(* Logix 5000 AddOnInstructionDefinition export YAI_Assy_72_73_120_EIP_Hz; software revision 21.03 *)

ADD_ON_INSTRUCTION YAI_Assy_72_73_120_EIP_Hz   (* revision 1.0, vendor Yaskawa America, Inc. *)
// YAI Assembly 72/73 and 120
// Help:
// This add-on instruction is for use with input assemblie 72/73 and output assemblies 120.
// Node_Input_Assy is defined as the node's input assembly integer array.
// Node_Output_Assy is defined as the node's output assembly integer array.
// Torque limit/reference, torque compensation and torque output variables are only available with A1000.
VAR_IN_OUT
   Node_Input_Assy : AB:ETHERNET_MODULE_INT_6Bytes:I:0; {required}   // Input assembly words
   Node_Output_Assy : AB:ETHERNET_MODULE_INT_24Bytes:O:0; {required}   // Output assembly words
END_VAR
VAR_INPUT
   RunFwd : BOOL; {visible}   // Forward run command
   RunRev : BOOL; {visible}   // Reverse run command
   MFI_3 : BOOL; {visible}   // Multi-function input 3
   MFI_4 : BOOL; {visible}   // Multi-function input 4
   MFI_5 : BOOL; {visible}   // Multi-function input 5
   MFI_6 : BOOL; {visible}   // Multi-function input 6
   MFI_7 : BOOL; {visible}   // Multi-function input 7
   MFI_8 : BOOL; {visible}   // Multi-function input 8
   External_Fault : BOOL;   // External fault command (EF0)
   FaultReset : BOOL; {visible}   // Fault reset command
   MFO_1 : BOOL; {visible}   // Multi-function output (M1-M2 for A/P1000, MA/MB/MC for V1000)
   MFO_2 : BOOL; {visible}   // Multi-function output (M3-M4 for A/P1000, P1 for V1000)
   MFO_3 : BOOL; {visible}   // Multi-function output (M5-M6 for A/P1000, P2 for V1000)
   Freq_Ref : REAL; {visible}   // Frequency reference command in Hz (xx.xx resolution)
   Digital_Output_Fault_Enable : BOOL;   // Bit to enable control of fault output relay over the network
   Custom_Out_1 : INT;
   Custom_Out_2 : INT;
   Custom_Out_3 : INT;
   Custom_Out_4 : INT;
   Custom_Out_5 : INT;
   Custom_Out_6 : INT;
   Custom_Out_7 : INT;
   Custom_Out_8 : INT;
   Custom_Out_9 : INT;
   Custom_Out_10 : INT;
END_VAR
VAR_OUTPUT
   Faulted : BOOL; {access Read Only, visible}   // Drive faulted status bit
   Output_Freq : REAL; {access Read Only, visible}   // Drive output frequency in Hz (xx.xx resolution)
   RunningFwd : BOOL; {access Read Only, visible}   // Drive running forward status bit
   Faulted1 : BOOL; {access Read Only, visible}   // Drive faulted status bit
   NetCtrlStatus : BOOL; {access Read Only, visible}   // Drive network run source status bit (1 = source coming from network)
   NetRefStatus : BOOL; {access Read Only, visible}   // Drive network reference status bit (1 = reference coming from network)
   Output_Freq1 : REAL; {access Read Only, visible}   // Drive output frequency in Hz (xx.xx resolution)
   Ready : BOOL; {access Read Only, visible}   // Drive ready status bit
   RunningFwd1 : BOOL; {access Read Only, visible}   // Drive running forward status bit
   RunningRev : BOOL; {access Read Only, visible}   // Drive running reverse status bit
   Torque_Actual : REAL; {access Read Only, visible}   // Drive torque output in engineering units.
   Warning : BOOL; {access Read Only, visible}   // Drive warning (alarm) status bit
   At_Speed : BOOL; {access Read Only, visible}   // Drive at commanded speed status bit
   Drive_State : INT; {access Read Only}   // Drive Status - Refer to class 0x29, Instance 0x1, Attribute 0x6 for details
END_VAR
VAR_INPUT
   Motor_Rated_Torq : REAL := 100.0; {visible}   // Motor rated torque (Engineering units)
END_VAR
VAR
   FRef_Convert : DINT;
   FOut_Convert : REAL;
   FOut_Temp : REAL;
   TRef_Convert : INT;
   TComp_Convert : INT;
   TOut_Convert : REAL;
   TOut_Temp : REAL;
   IOut_Temp : REAL;
   IOut_Convert : REAL;
   AO1_Convert : INT;
   AO2_Convert : INT;
   Motor_Speed_Temp : REAL;
   Motor_Speed_Convert : REAL;
   Freq_Cmd_Temp : REAL;
   Freq_Cmd_Convert : REAL;
   AI1_Temp : REAL;
   AI1_Convert : REAL;
   AI2_Temp : REAL; {access None}
   AI2_Convert : REAL; {access None}
   AI3_Temp : REAL; {access None}
   AI3_Convert : REAL; {access None}
   DriveStatusTempBits : INT;
   Tout_Convert_Temp : REAL;
END_VAR

ROUTINE Logic   (* ladder *)
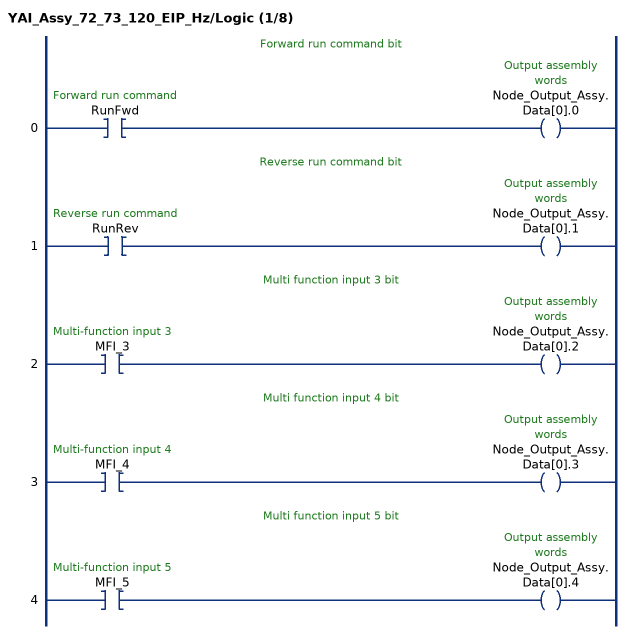
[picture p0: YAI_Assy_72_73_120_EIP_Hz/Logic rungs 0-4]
   // Forward run command bit
   0: XIC(RunFwd)OTE(Node_Output_Assy.Data[0].0);
   // Reverse run command bit
   1: XIC(RunRev)OTE(Node_Output_Assy.Data[0].1);
   // Multi function input 3 bit
   2: XIC(MFI_3)OTE(Node_Output_Assy.Data[0].2);
   // Multi function input 4 bit
   3: XIC(MFI_4)OTE(Node_Output_Assy.Data[0].3);
   // Multi function input 5 bit
   4: XIC(MFI_5)OTE(Node_Output_Assy.Data[0].4);
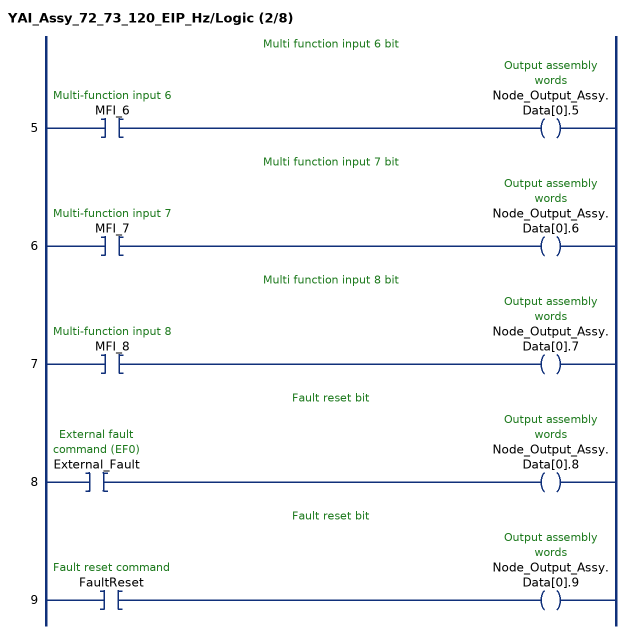
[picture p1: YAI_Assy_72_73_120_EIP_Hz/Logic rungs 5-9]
   // Multi function input 6 bit
   5: XIC(MFI_6)OTE(Node_Output_Assy.Data[0].5);
   // Multi function input 7 bit
   6: XIC(MFI_7)OTE(Node_Output_Assy.Data[0].6);
   // Multi function input 8 bit
   7: XIC(MFI_8)OTE(Node_Output_Assy.Data[0].7);
   // Fault reset bit
   8: XIC(External_Fault)OTE(Node_Output_Assy.Data[0].8);
   // Fault reset bit
   9: XIC(FaultReset)OTE(Node_Output_Assy.Data[0].9);
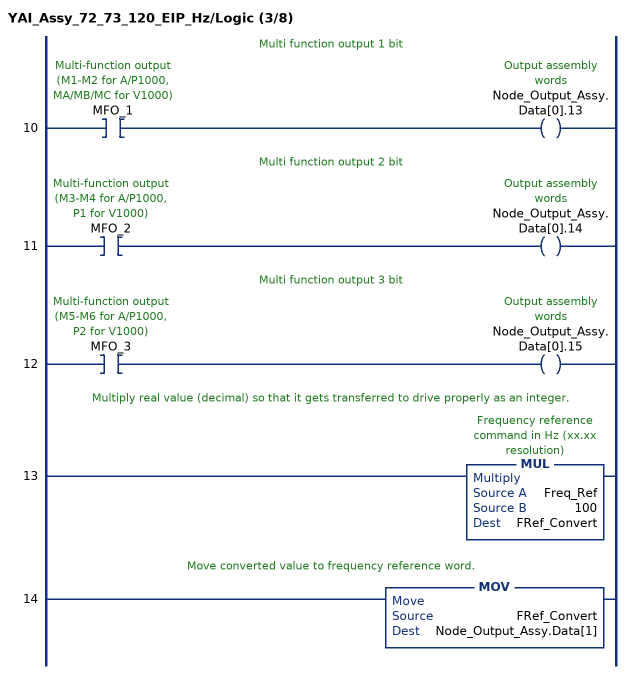
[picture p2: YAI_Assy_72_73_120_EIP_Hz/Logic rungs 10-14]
   // Multi function output 1 bit
   10: XIC(MFO_1)OTE(Node_Output_Assy.Data[0].13);
   // Multi function output 2 bit
   11: XIC(MFO_2)OTE(Node_Output_Assy.Data[0].14);
   // Multi function output 3 bit
   12: XIC(MFO_3)OTE(Node_Output_Assy.Data[0].15);
   // Multiply real value (decimal) so that it gets transferred to drive properly as an integer.
   13: MUL(Freq_Ref,100,FRef_Convert);
   // Move converted value to frequency reference word.
   14: MOV(FRef_Convert,Node_Output_Assy.Data[1]);
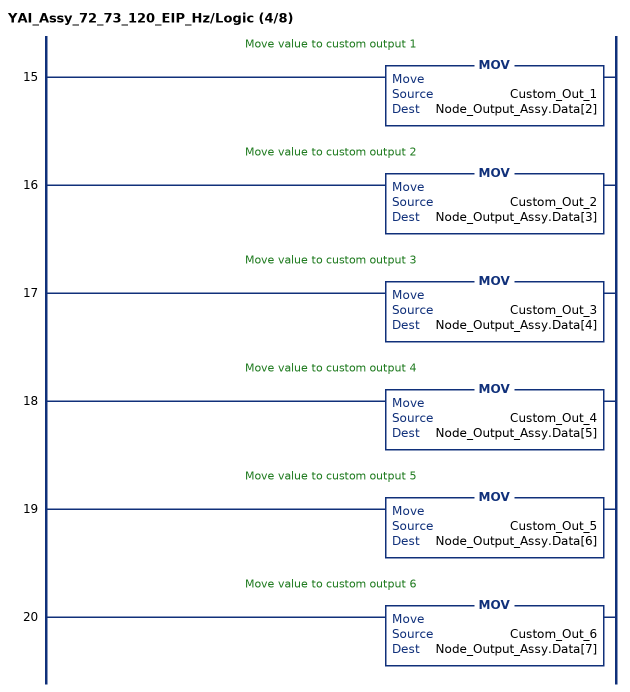
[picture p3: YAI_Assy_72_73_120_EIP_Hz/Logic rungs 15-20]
   // Move value to custom output 1
   15: MOV(Custom_Out_1,Node_Output_Assy.Data[2]);
   // Move value to custom output 2
   16: MOV(Custom_Out_2,Node_Output_Assy.Data[3]);
   // Move value to custom output 3
   17: MOV(Custom_Out_3,Node_Output_Assy.Data[4]);
   // Move value to custom output 4
   18: MOV(Custom_Out_4,Node_Output_Assy.Data[5]);
   // Move value to custom output 5
   19: MOV(Custom_Out_5,Node_Output_Assy.Data[6]);
   // Move value to custom output 6
   20: MOV(Custom_Out_6,Node_Output_Assy.Data[7]);
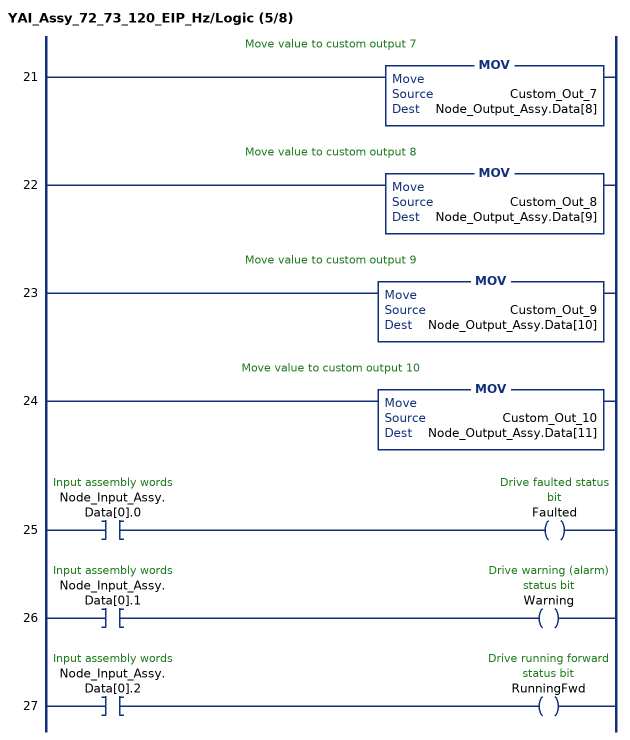
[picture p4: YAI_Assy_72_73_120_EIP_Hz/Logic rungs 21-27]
   // Move value to custom output 7
   21: MOV(Custom_Out_7,Node_Output_Assy.Data[8]);
   // Move value to custom output 8
   22: MOV(Custom_Out_8,Node_Output_Assy.Data[9]);
   // Move value to custom output 9
   23: MOV(Custom_Out_9,Node_Output_Assy.Data[10]);
   // Move value to custom output 10
   24: MOV(Custom_Out_10,Node_Output_Assy.Data[11]);
   25: XIC(Node_Input_Assy.Data[0].0)OTE(Faulted);
   26: XIC(Node_Input_Assy.Data[0].1)OTE(Warning);
   27: XIC(Node_Input_Assy.Data[0].2)OTE(RunningFwd);
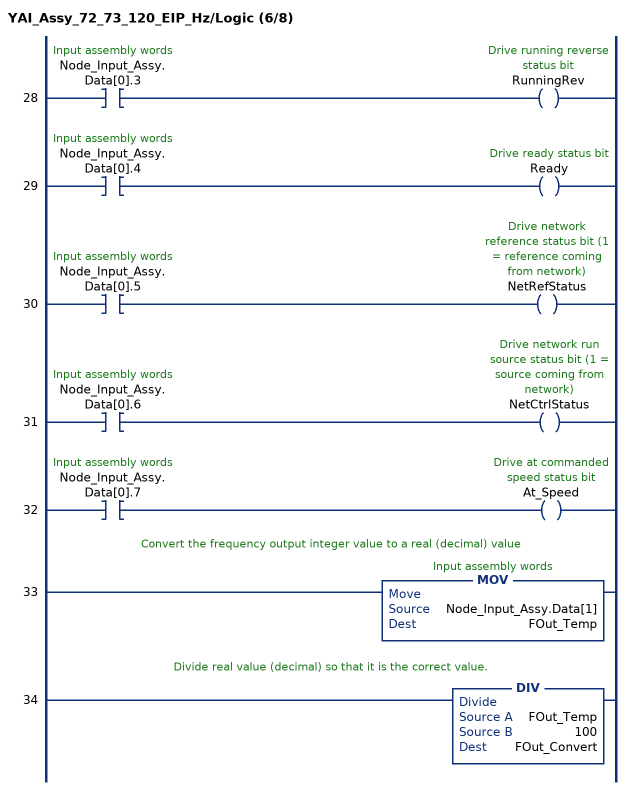
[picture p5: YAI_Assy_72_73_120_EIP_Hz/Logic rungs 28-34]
   28: XIC(Node_Input_Assy.Data[0].3)OTE(RunningRev);
   29: XIC(Node_Input_Assy.Data[0].4)OTE(Ready);
   30: XIC(Node_Input_Assy.Data[0].5)OTE(NetRefStatus);
   31: XIC(Node_Input_Assy.Data[0].6)OTE(NetCtrlStatus);
   32: XIC(Node_Input_Assy.Data[0].7)OTE(At_Speed);
   // Convert the frequency output integer value to a real (decimal) value
   33: MOV(Node_Input_Assy.Data[1],FOut_Temp);
   // Divide real value (decimal) so that it is the correct value.
   34: DIV(FOut_Temp,100,FOut_Convert);
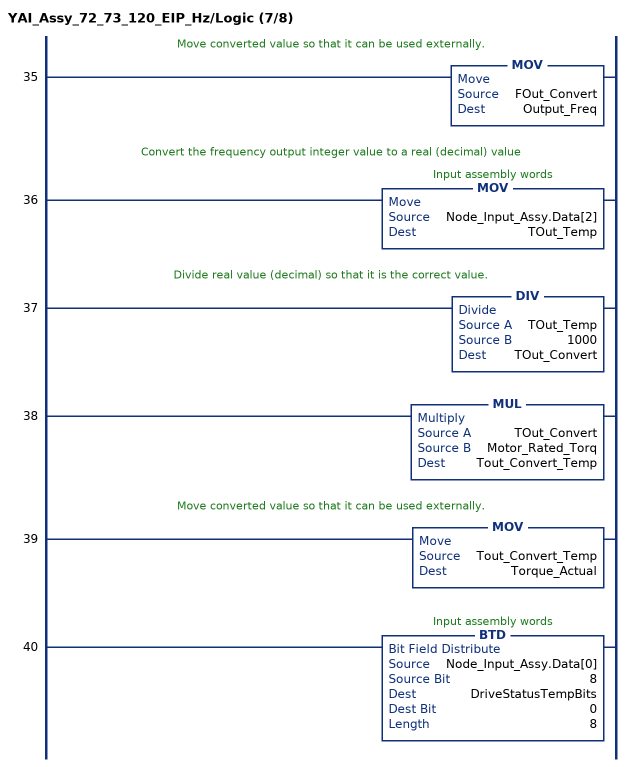
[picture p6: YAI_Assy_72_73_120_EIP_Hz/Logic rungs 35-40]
   // Move converted value so that it can be used externally.
   35: MOV(FOut_Convert,Output_Freq);
   // Convert the frequency output integer value to a real (decimal) value
   36: MOV(Node_Input_Assy.Data[2],TOut_Temp);
   // Divide real value (decimal) so that it is the correct value.
   37: DIV(TOut_Temp,1000,TOut_Convert);
   38: MUL(TOut_Convert,Motor_Rated_Torq,Tout_Convert_Temp);
   // Move converted value so that it can be used externally.
   39: MOV(Tout_Convert_Temp,Torque_Actual);
   40: BTD(Node_Input_Assy.Data[0],8,DriveStatusTempBits,0,8);
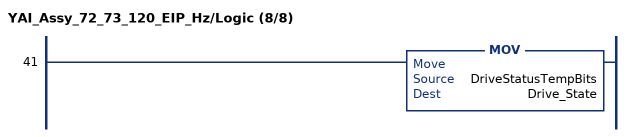
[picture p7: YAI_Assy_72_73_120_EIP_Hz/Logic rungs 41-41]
   41: MOV(DriveStatusTempBits,Drive_State);
END_ROUTINE
END_ADD_ON_INSTRUCTION
